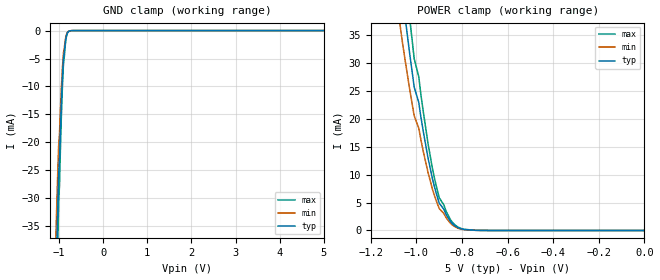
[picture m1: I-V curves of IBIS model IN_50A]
| TEXAS INSTRUMENTS INCORPORATED
| Standard Linear and Logic Group / High Volume Linear
| IBIS Model of TPD1E05U06
| Single Channel ESD Protection Device
| This file contains package information for the following:
|  QFN 2-pin (DPY) package as [Component] TPD1E05U06_DPY
| This device can be powered at the following Vccs:
|  5 volt Vcc
| This file provides unique models under the [Model Selector] for each Vcc.
| For operation at a specific Vcc, select the appropriate model after each
| [Model Selector] keyword.
[IBIS Ver]   3.2
[Comment char]  |_char
[File Name]   tpd1e05u06.ibs
[File Rev]   1.1
[Date]   12/10/2015
[Source]   Data created from TI-SPICE simulations at TI-SLL/HVL.
   The following is an IBIS list for the TPD1E05U06.
   Please contact sllibis@ti.com with questions and
   comments concerning SLL IBIS models.
[Notes]   Revision_History:
|  Rev 1.1   12/10/2015
|  - c comp values revised per PL's request
|  Rev 1.0 October 25, 2012
[Disclaimer]
| This model is designed as an aid for customers of Texas Instruments.
| TI and its licensors and suppliers make no warranties, either expressed
| or implied, with respect to this  model, including the warranties of
| merchantability or fitness for a particular purpose. The model is
| provided solely on an "as is" basis. The entire risk as to its quality
| and performance is with the customer.
[Copyright]
| (C) Copyright 2012 Texas Instruments Incorporated. All rights reserved.
| Component TPD1E05U06_DPY 2-PIN QFN
[Component]   TPD1E05U06_DPY
[Manufacturer]   Texas Instruments, Inc.
[Package]
|   typ   min   max
R_pkg   6.000e-02   5.900e-02   6.100e-02
L_pkg   5.003e-10   4.430e-10   5.015e-10
C_pkg   2.000e-14   1.990e-14   2.010e-14
[Pin]   signal_name   model_name   R_pin   L_pin   C_pin
1   1   IN_50A   6.100e-02   4.430e-10   1.990e-14
2   2   GND   6.100e-02   4.430e-10   1.990e-14
| Models and submodels in the file (1): IN_50A (Input)
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| Model IN
[Model]   IN_50A
Model_type  Input
Vinl=0
Vinh=5
| variable   typ   min   max
C_comp   0.40pF   0.30pF   0.70pF
[Temperature Range]   40   100   -40
| Ambient temperature   25   85   -40
[Voltage range]   5   5   5
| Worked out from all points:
|   GND clamp passes 1 mA (typ) near -0.84 V on its own axis
|   POWER clamp passes 1 mA (typ) near -0.84 V on its own axis
[GND Clamp]
| IN_50A
| Voltage   I(typ)   I(min)   I(max)
-5V       -1.23A     -985mA     -1.48A
-1.07V    -45.16mA   -36.1mA    -54.2mA
-1.05V    -38.18mA   -30.5mA    -45.8mA
-1.03V    -31.67mA   -25.3mA    -38mA
-1.02V    -28.68mA   -22.9mA    -34.4mA
-1.01V    -25.62mA   -20.5mA    -30.7mA
-990mV    -22.9mA    -18.3mA    -27.5mA
-950mV    -13.12mA   -10.5mA    -15.7mA
-900mV    -4.871mA   -3.9mA     -5.84mA
-850mV    -1.552mA   -1.24mA    -1.86mA
-790mV    -170.1uA   -136uA     -204uA
5V        247pA      198pA      296pA
[POWER Clamp]
| IN_50A
|Voltage   I(typ)   I(min)   I(max)
-5V       1.23A      985mA      1.48A
-1.07V    45.16mA    36.1mA     54.2mA
-1.05V    38.18mA    30.5mA     45.8mA
-1.03V    31.67mA    25.3mA     38mA
-1.02V    28.68mA    22.9mA     34.4mA
-1.01V    25.62mA    20.5mA     30.7mA
-990mV    22.9mA     18.3mA     27.5mA
-950mV    13.12mA    10.5mA     15.7mA
-920mV    7.63mA     6.1mA      9.16mA
-900mV    4.871mA    3.9mA      5.84mA
-830mV    797.3uA    638uA      957uA
0V        0A         0A         0A
